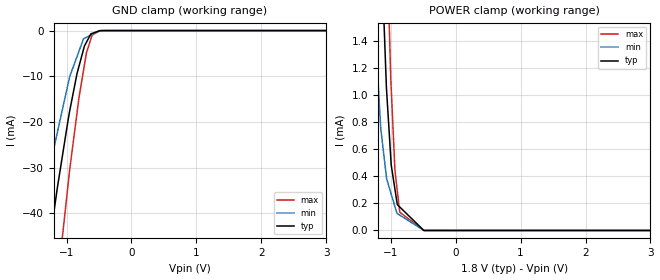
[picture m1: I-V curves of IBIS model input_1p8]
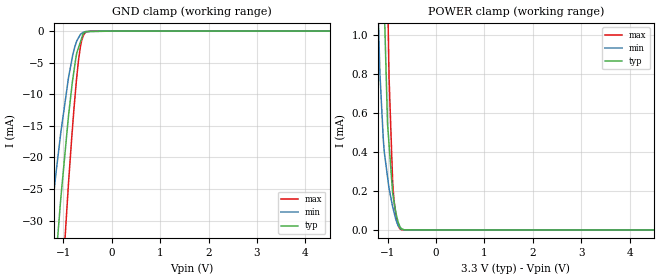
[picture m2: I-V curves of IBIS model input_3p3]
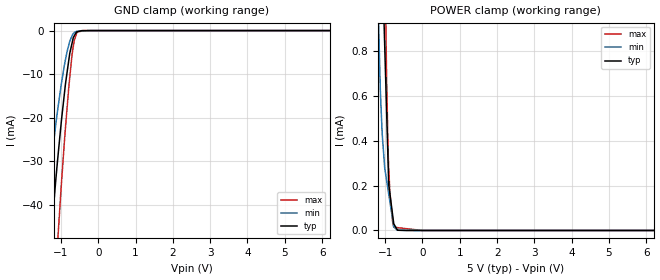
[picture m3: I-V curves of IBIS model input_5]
|Texas Instruments Incorporated
|2.7V~5.5V, 16 Bit 1MSPS Serial ADC
| Marketing part#   Digital Voltage Range   Package-type   #pins
| ADS8329IBPW   1.65V - 5.5V   TSSOP   16
| ADS8329IBPWG4   1.65V - 5.5V   TSSOP   16
| ADS8329IBPWR   1.65V - 5.5V   TSSOP   16
| ADS8329IBPWRG4   1.65V - 5.5V   TSSOP   16
| ADS8329IPW   1.65V - 5.5V   TSSOP   16
| ADS8329IPWG4   1.65V - 5.5V   TSSOP   16
| ADS8329IPWR   1.65V - 5.5V   TSSOP   16
| ADS8329IPWRG4   1.65V - 5.5V   TSSOP   16
| ADS8329IBRSAR   1.65V - 5.5V   QFN   16
| ADS8329IBRSARG4   1.65V - 5.5V   QFN   16
| ADS8329IBRSAT   1.65V - 5.5V   QFN   16
| ADS8329IBRSATG4   1.65V - 5.5V   QFN   16
| ADS8329IRSAR   1.65V - 5.5V   QFN   16
| ADS8329IRSARG4   1.65V - 5.5V   QFN   16
| ADS8329IRSAT   1.65V - 5.5V   QFN   16
| ADS8329IRSATG4   1.65V - 5.5V   QFN   16
[IBIS Ver]   3.2
[File name]   ads8329.ibs
|SIMDE Ver   V3.0 - 201101 - Build 453
[File Rev]   1.0
[Date]   4/29/2011
[Source]
| Texas Instruments Incorporated.
| Analog-eLab Design Center, HPA
| 12500 TI Blvd
| Dallas, TX -75243
| e-mail: elab_ibis@list.ti.com
| -Model generated from simulations in TISPICE
[Notes]   Revision History:
| Rev 1.0: 4/29/2011
| - Initial version of the model
| - Model generated from simulations in TISPICE
| - Model matched to SPICE simulation
| - Model names with a trailing 1p8 contains the model for
|   1.8V [1.65V and 1.96V].
| - Model names with a trailing 3p3 contains the model for
|   3.3V [3.0V and 3.6V].
| - Model names with trailing 5 contains
|   the model for 5.0V [4.5V and 5.5V] operation.
| - C_comp although listed in numerical order of value are
|   obtained from varying PVT conditions. For PVT conditions for
|   each specific value refer the buffer description under
|   respective [Model]. IBIS model user is responsible for using
|   appropriate C_comp to simulate for Signal Integrity.
| - This part is relative of ADS8327
[Disclaimer]
| This model is designed as an aid for customers of Texas Instruments.
| TI and its licensors and suppliers make no warranties, either expressed
| or implied, with respect to this  model, including the warranties of
| merchantability or fitness for a particular purpose. The model is
| provided solely on an "as is" basis. The entire risk as to its quality
| and performance is with the customer.
[Copyright]
 (C) Copyright 2011 Texas Instruments Incorporated.All rights reserved.
|   ADS8329PW
[Component]   ADS8329PW
[Manufacturer]   TI
[Package]   |16 TSSOP - PW package
|   typ   min   max
R_pkg   0.17607   0.15537   0.21753
L_pkg   2.43370nH   2.20397nH   3.33174nH
C_pkg   0.44719pF   0.43609pF   0.50154pF
[Pin]  signal_name   model_name   R_pin   L_pin   C_pin
1   +VA   POWER   0.07656   2.68034nH  0.55807pF
2   RESERVED   TERM   0.18387   2.44521nH  0.43752pF
3   +IN   TERM   0.15983   2.24102nH  0.44342pF
4   -IN   TERM   0.15537   2.20397nH  0.44187pF
5   AGND   GND   0.05746   1.76459nH  0.49499pF
6   REF-   TERM   0.16557   2.28939nH  0.44710pF
7   REF+   TERM   0.18345   2.44488nH  0.43609pF
8   NC   NC   0.01109   1.86891nH  0.43090pF
9   _CONVST   input   0.21753   3.33174nH  0.50154pF
10   EOC/_INT/CDI   io   0.19564   2.54541nH  0.44055pF
11   FS/_CS   input   0.16494   2.28442nH  0.44487pF
12   SDI   input   0.15782   2.22466nH  0.44218pF
13   SDO   sdo   0.16241   2.26113nH  0.44399pF
14   BDGND   GND   0.08607   1.97322nH  0.47016pF
15   SCLK   input   0.19036   2.49888nH  0.43998pF
16   +VBD   POWER   0.10998   2.81120nH  0.53392pF
|   ADS8329RSA
[Component]   ADS8329RSA
[Manufacturer]   TI
[Package]   |16 QFN   - RSA package
|   typ   min   max
R_pkg   0.066285   0.05989   0.07105
L_pkg   1.050497nH   0.93922nH   1.12758nH
C_pkg   0.15367pF   0.14322pF   0.16581pF
[Pin]  signal_name   model_name   R_pin   L_pin   C_pin
1   REF+   TERM   0.06343   1.00437nH  0.14519pF
2   NC   NC   0.00077   0.12730nH  0.10311pF
3   _CONVST   input   0.06559   1.03450nH  0.16110pF
4   EOC/_INT/CDI   io   0.06320   1.00058nH  0.14575pF
5   FS/_CS   input   0.07073   1.12267nH  0.15243pF
6   SDI   input   0.06817   1.07390nH  0.16369pF
7   SDO   sdo   0.07015   1.10578nH  0.16581pF
8   BDGND   GND   0.03602   0.84904nH  0.17939pF
9   SCLK   input   0.06063   0.95120nH  0.14366pF
10   +VBD   POWER   0.03041   0.64603nH  0.18521pF
11   +VA   POWER   0.02066   0.56224nH  0.20728pF
12   RESERVED   TERM   0.05989   0.93922nH  0.14322pF
13   +IN   TERM   0.06886   1.08873nH  0.15083pF
14   -IN   TERM   0.06744   1.06081nH  0.16356pF
15   AGND   GND   0.02332   0.65734nH  0.22188pF
16   REF-   TERM   0.07105   1.12758nH  0.15513pF
|   Model Selectors
[Model Selector] input
input_1p8  1.8V digital input
input_3p3  3.3V digital input
input_5   5.0V digital input
[Model Selector] io
io_1p8   1.8V  digital io
io_3p3   3.3V  digital io
io_5   5.0V  digital io
[Model Selector] sdo
sdo_1p8   1.8V  digital 3-state output
sdo_3p3   3.3V  digital 3-state output
sdo_5   5.0V  digital 3-state output
[Model Selector] TERM
TERM_1p8  1.8V nominal termination
TERM_3p3  3.3V nominal termination
TERM_5   5.0V nominal termination
[Model]  TERM_1p8
Model_type Terminator
C_comp   1.0e-20F  1.0e-20F  1.0e-20F
|   typ   min   max
[Voltage Range]   1.8V   1.65V   1.96V
[POWER Clamp Reference]   1.8V   1.65V   1.96V
[GND Clamp Reference]   0V   0V   0V
|Ambient Temperature   25   85   -40
|Junction Temperature
[Temperature Range]   28   88   -40
[Model]  TERM_3p3
Model_type Terminator
C_comp   1.0e-20F  1.0e-20F  1.0e-20F
|   typ   min   max
[Voltage Range]   3.3V   3.0V   3.6V
[POWER Clamp Reference]   3.3V   3.0V   3.6V
[GND Clamp Reference]   0V   0V   0V
|Ambient Temperature   25   85   -40
|Junction Temperature
[Temperature Range]   28   88   -40
[Model]  TERM_5
Model_type Terminator
C_comp   1.0e-20F  1.0e-20F  1.0e-20F
|   typ   min   max
[Voltage Range]   5.0V   4.5V   5.5V
[POWER Clamp Reference]   5.0V   4.5V   5.5V
[GND Clamp Reference]   0V   0V   0V
|Ambient Temperature   25   85   -40
|Junction Temperature
[Temperature Range]   28   88   -40
| Models and submodels in the file (12): input_1p8 (Input), input_3p3 (Input), input_5 (Input), io_1p8 (I/O), io_3p3 (I/O), io_5 (I/O), sdo_1p8 (3-state), sdo_3p3 (3-state), sdo_5 (3-state), TERM_1p8 (Terminator), TERM_3p3 (Terminator), TERM_5 (Terminator)
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|   input_1p8 Model
[Model]   input_1p8
Model_type   Input
Vinl = 0.63
Vinh = 1.17
|   typ   min   max
|   (nom PVT)   (Fast PVT)   (slow PVT)
|C_comp from frequency sweep method(F=50MHz)
C_comp   1.266e-12   1.220e-12   1.302e-12
|C_comp from LC tank measurement(L=1nH)
|C_comp   1.129e-12   1.091e-12   1.183e-12
|Resonant Frequency(Hz)   4.740e+09   4.820e+09   4.630e+09
| Where nom  PVT is Nominal Process,  1.8V,  28C
|   Fast PVT is Strong Process,   1.96V,  -40C
|   Slow PVT is Weak Process,   1.65V,  88C
[Model Spec]
Vinl   0.63   0.58   0.68
Vinh   1.17   1.07   1.27
[Voltage Range]   1.8   1.65   1.96
|Ambient Temperature   25   85   -40
|Junction Temperature
[Temperature Range]   28   88   -40
[Power Clamp Reference]   1.8   1.65   1.96
[GND Clamp Reference]   0   0   0
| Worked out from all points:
|   GND clamp passes 1 mA (typ) near -0.64 V on its own axis
|   POWER clamp passes 1 mA (typ) near -1.06 V on its own axis
[GND Clamp]
|   Voltage   I(typ)   I(min)   I(max)
-1.8V     -107.8mA   -73.25mA   -158.4mA
-1.65V    -90.51mA   -61.18mA   -134.6mA
-1.332V   -53.84mA   -35.57mA   -84.15mA
-1.267V   -47mA      -30.35mA   -74.13mA
-1.103V   -31.02mA   -19.86mA   -50.33mA
-975.6mV  -19.56mA   -11.66mA   -33.63mA
-838.8mV  -9.437mA   -5.712mA   -18.07mA
-737.6mV  -4.083mA   -1.797mA   -8.651mA
-693.8mV  -2.571mA   -1.486mA   -4.916mA
-624.6mV  -717.3uA   -992.7uA   -1.83mA
-456.7mV  -12.01uA   -10.57uA   -10.57uA
3.6V      0A         0A         0A
[POWER Clamp]
|   Voltage   I(typ)   I(min)   I(max)
-1.8V     13.74mA    9.485mA    18.5mA
-1.239V   3.538mA    1.477mA    5.738mA
-1.155V   2.216mA    768.2uA    3.991mA
-1.103V   1.545mA    549.8uA    2.922mA
-1.063V   1.028mA    381.9uA    2.217mA
-1.002V   558uA      283.7uA    1.164mA
-991.8mV  482.8uA    268uA      1.048mA
-934.9mV  305.7uA    176.4uA    444.6uA
-898.2mV  191.3uA    125.1uA    292uA
-860.4mV  173.6uA    113.6uA    135uA
-489.6mV  0A         369.6nA    565.8nA
3.6V      0A         0A         0A
|   input_3p3 Model
[Model]   input_3p3
Model_type   Input
Vinl = 1.15
Vinh = 2.14
|   typ   min   max
|   (nom PVT)   (Fast PVT)   (slow PVT)
|C_comp from frequency sweep method(F=50MHz)
|C_comp   1.190e-12   1.134e-12   1.234e-12
|C_comp from LC tank measurement(L=1nH)
C_comp   1.078e-12   1.039e-12   1.129e-12
|Resonant Frequency(Hz)   4.850e+09   4.940e+09   4.740e+09
| Where nom  PVT is Nominal Process,  3.3V,  28C
|   Fast PVT is Strong Process,   3.6V,  -40C
|   Slow PVT is Weak Process,   3V,  88C
[Model Spec]
Vinl   1.15   1.05   1.26
Vinh   2.14   1.95   2.34
[Voltage Range]   3.3   3   3.6
|Ambient Temperature   25   85   -40
|Junction Temperature
[Temperature Range]   28   88   -40
[Power Clamp Reference]   3.3   3   3.6
[GND Clamp Reference]   0   0   0
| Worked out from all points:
|   GND clamp passes 1 mA (typ) near -0.62 V on its own axis
|   POWER clamp passes 1 mA (typ) near -1.05 V on its own axis
[GND Clamp]
|   Voltage   I(typ)   I(min)   I(max)
-3.3V     -298.8mA   -220.8mA   -406.2mA
-1.439V   -65.52mA   -43.56mA   -100.7mA
-1.245V   -44.76mA   -28.74mA   -70.74mA
-1.152V   -35.69mA   -22.26mA   -57.16mA
-1.059V   -26.76mA   -16.27mA   -44.43mA
-1.019V   -23.42mA   -14.05mA   -38.93mA
-897.6mV  -13.49mA   -7.421mA   -24.21mA
-818.4mV  -8.163mA   -4.174mA   -15.73mA
-694.8mV  -2.745mA   -1.135mA   -4.979mA
-591mV    -353.4uA   -186.2uA   -741uA
-439.2mV  -78.48uA   -40.31uA   -5.555uA
6.6V      0A         0A         0A
[POWER Clamp]
|   Voltage   I(typ)   I(min)   I(max)
-3.3V     43.07mA    34.83mA    54.13mA
-1.211V   3.046mA    1.261mA    5.284mA
-1.164V   2.375mA    827uA      4.3mA
-1.089V   1.315mA    458.5uA    2.733mA
-1.055V   1.008mA    371uA      2.019mA
-1.003V   546.1uA    273.1uA    1.247mA
-896.4mV  188.2uA    118.2uA    239.9uA
-860.4mV  129.5uA    82.19uA    134.9uA
-813.6mV  69.71uA    40.8uA     54.22uA
-766.8mV  29.28uA    16.98uA    12.79uA
-709.2mV  4.986uA    4.597uA    1.015uA
6.6V      0A         0A         0A
|   input_5 Model
[Model]   input_5
Model_type   Input
Vinl = 1.75
Vinh = 3.25
|   typ   min   max
|   (nom PVT)   (Fast PVT)   (slow PVT)
|C_comp from frequency sweep method(F=50MHz)
|C_comp   1.138e-12   1.109e-12   1.176e-12
|C_comp from LC tank measurement(L=1nH)
C_comp   1.039e-12   1.002e-12   1.082e-12
|Resonant Frequency(Hz)   4.940e+09   5.030e+09   4.840e+09
| Where nom  PVT is Nominal Process,  5V,  28C
|   Fast PVT is Strong Process,   5.5V,  -40C
|   Slow PVT is Weak Process,   4.5V,  88C
[Model Spec]
Vinl   1.75   1.57   1.92
Vinh   3.25   2.92   3.57
[Voltage Range]   5   4.5   5.5
|Ambient Temperature   25   85   -40
|Junction Temperature
[Temperature Range]   28   88   -40
[Power Clamp Reference]   5   4.5   5.5
[GND Clamp Reference]   0   0   0
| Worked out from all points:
|   GND clamp passes 1 mA (typ) near -0.63 V on its own axis
|   POWER clamp passes 1 mA (typ) near -1.04 V on its own axis
[GND Clamp]
|   Voltage   I(typ)   I(min)   I(max)
-5V       -519.6mA   -396mA     -686mA
-1.565V   -79.89mA   -53.97mA   -120.4mA
-1.375V   -58.48mA   -38.5mA    -90.46mA
-1.226V   -43.19mA   -27.76mA   -67.98mA
-1.095V   -30.01mA   -18.57mA   -49.08mA
-1.022V   -23.54mA   -14.02mA   -39.41mA
-907.5mV  -14.35mA   -7.892mA   -25.32mA
-786.5mV  -6.525mA   -3.163mA   -12.58mA
-693mV    -2.489mA   -998.5uA   -4.86mA
-643.5mV  -1.209mA   -464uA     -2.209mA
-585mV    -304uA     -166.9uA   -748.3uA
10V       0A         0A         0A
[POWER Clamp]
|   Voltage   I(typ)   I(min)   I(max)
-5V       76.86mA    64.15mA    94.96mA
-1.183V   2.644mA    969.1uA    4.554mA
-1.08V    1.211mA    430.1uA    2.483mA
-1.012V   822.9uA    277.5uA    1.325mA
-1.001V   756.8uA    265.1uA    1.157mA
-962.5mV  535.2uA    223.7uA    683.9uA
-924mV    313.6uA    182.4uA    372.9uA
-905mV    204.3uA    161.9uA    277.3uA
-874.5mV  164.9uA    129.2uA    169.7uA
-770mV    29.83uA    16.87uA    14.44uA
-670.5mV  1.356uA    960.4nA    12.58uA
10V       0A         0A         0A
